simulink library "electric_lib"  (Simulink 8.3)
settings: Solver=ode45  StartTime=0.0  StopTime=10.0  RelTol=1e-3
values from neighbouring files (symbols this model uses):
  battery = class_REVS_battery    [class_REVS_electric.m]
  electric = class_REVS_electric(engine)    [electric_standard_car.m]
undefined symbols (not defined in the file or in its folder): alternator, converter, ConverterEfficiency_norm, emachine, starter
libraries: simulink x14, general_lib x14, audit_lib x9, electric_lib x5

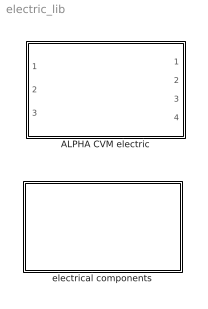
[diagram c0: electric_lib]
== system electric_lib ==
  ALPHA CVM electric : Subsystem  VariantControl=variants_electric_ALPHA
  electrical components : Subsystem

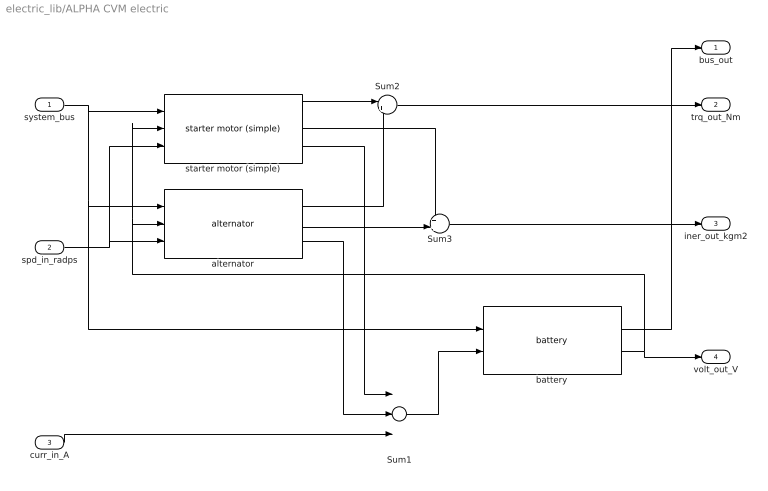
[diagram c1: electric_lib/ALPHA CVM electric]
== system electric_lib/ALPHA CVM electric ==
  system_bus : Inport
  spd_in_radps : Inport  Port=2
  curr_in_A : Inport  Port=3
  Sum1 : Sum  Inputs=+++
  Sum2 : Sum  Inputs=|++
  Sum3 : Sum  Inputs=++|
  alternator : electric_lib/electrical components/alternator  base_name=alternator  alternator=electric.alternator
  battery : electric_lib/electrical components/battery  BaseName=battery  battery=electric.battery
  starter motor (simple) : electric_lib/electrical components/starter motor (simple)  base_name=starter  starter=electric.starter
  bus_out : Outport
  trq_out_Nm : Outport  Port=2
  iner_out_kgm2 : Outport  Port=3
  volt_out_V : Outport  Port=4
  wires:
  spd_in_radps/1 -> alternator/3, starter motor (simple)/3
  Sum2/1 -> trq_out_Nm/1
  Sum3/1 -> iner_out_kgm2/1
  system_bus/1 -> battery/1, alternator/1, starter motor (simple)/1
  battery/2 -> volt_out_V/1, starter motor (simple)/2, alternator/2
  alternator/2 -> Sum3/2
  starter motor (simple)/2 -> Sum3/1
  alternator/1 -> Sum2/2
  starter motor (simple)/1 -> Sum2/1
  battery/1 -> bus_out/1
  starter motor (simple)/3 -> Sum1/1
  alternator/3 -> Sum1/2
  Sum1/1 -> battery/2
  curr_in_A/1 -> Sum1/3

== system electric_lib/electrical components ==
  alternator : Subsystem
  battery : Subsystem
  constant voltage power converter : Subsystem
  emachine : Subsystem
  starter motor (simple) : Subsystem
  thrushaft emachine : Subsystem
  variable voltage power converter : Subsystem

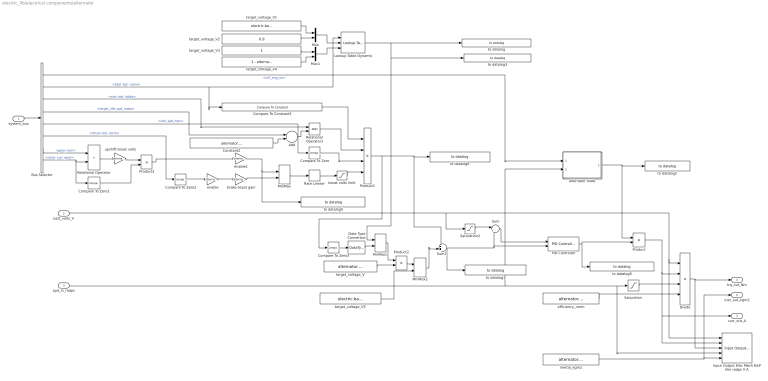
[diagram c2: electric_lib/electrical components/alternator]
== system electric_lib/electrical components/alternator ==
  system_bus : Inport
  batt_volts_V : Inport  Port=2
  spd_in_radps : Inport  Port=3
  Add : Sum
  Bus Selector : BusSelector  OutputSignals=powertrain.control.ctrl_eng_on,powertrain.signal4.batt_SoC_norm,powertrain.engine.eng_spd_radps,powertrain.engine.target_idle_spd_radps,vehicle.veh_spd_mps,driver.driver_brk_norm,powertrain.trans.ctrl.gear_num,powertrain.trans.ctrl.dct_core_ctrl.trans_curr_gear
  Compare To Constant2 : simulink/Logic and Bit Operations/Compare To Constant  relop=<=  const=alternator.regen_boost_max_battery_soc_norm  OutDataTypeStr=boolean  ZeroCross=off
  Compare To Zero{,1..3} (4 alike) : simulink/Logic and Bit Operations/Compare To Zero  relop=>  OutDataTypeStr=boolean  ZeroCross=off
  Constant2 : Constant  Value=alternator.regen_idle_speed_offset_radps
  Data Type Conversion : DataTypeConversion
  Divide : Product  Inputs=**//
  Input Output Elec Mech E&P Nm radps V A : audit_lib/Input Output Elec Mech E&P Nm radps V A  base_name=alternator  VerboseSignal=REVS.verbose
  Lookup Table Dynamic : simulink/Lookup Tables/Lookup Table Dynamic  LookUpMeth=Interpolation-Use End Values  OutDataTypeStr=double  OutputDataTypeScalingMode=Specify via dialog  OutDataType=fixdt('double')  OutScaling=2^-10  DoSatur=off
  MinMax : MinMax  Function=max  Inputs=2
  MinMax1 : MinMax  Function=max  Inputs=2
  MinMax2 : MinMax  Function=max  Inputs=2
  Mux : Mux  Inputs=2
  Mux1 : Mux  Inputs=2
  PID Controller : simulink/Continuous/PID Controller  Controller=PID  TimeDomain=Continuous-time  SampleTime=1  IntegratorMethod=Forward Euler  FilterMethod=Forward Euler  Form=Parallel  P=alternator.nominal_Kp * (1 + alternator.regen_Kp_multiplier*alternator.regen_enable)  I=alternator.nominal_Ki * (1 + alternator.regen_Ki_multiplier*alternator.regen_enable)  D=0  N=1  InitialConditionSource=internal  InitialConditionForIntegrator=0  InitialConditionForFilter=0  ExternalReset=falling  ZeroCross=off  LimitOutput=on  UpperSaturationLimit=0  LowerSaturationLimit=-alternator.max_current_A  LinearizeAsGain=on  AntiWindupMode=clamping  Kb=1  TrackingMode=off  Kt=1  PParamMin=[]  PParamMax=[]  IParamMin=[]  IParamMax=[]  DParamMin=[]  DParamMax=[]  NParamMin=[]  NParamMax=[]  KbParamMin=[]  KbParamMax=[]  KtParamMin=[]  KtParamMax=[]  POutMin=[]  POutMax=[]  IOutMin=[]  IOutMax=[]  DOutMin=[]  DOutMax=[]  NOutMin=[]  NOutMax=[]  KbOutMin=[]  KbOutMax=[]  KtOutMin=[]  KtOutMax=[]  IntegratorOutMin=[]  IntegratorOutMax=[]  FilterOutMin=[]  FilterOutMax=[]  SumOutMin=[]  SumOutMax=[]  SumI1OutMin=[]  SumI1OutMax=[]  SumI2OutMin=[]  SumI2OutMax=[]  SumI3OutMin=[]  SumI3OutMax=[]  SumDOutMin=[]  SumDOutMax=[]  SaturationOutMin=[]  SaturationOutMax=[]  IntegratorContinuousStateAttributes=''  IntegratorStateMustResolveToSignalObject=off  IntegratorRTWStateStorageClass=Auto  FilterContinuousStateAttributes=''  FilterStateMustResolveToSignalObject=off  FilterRTWStateStorageClass=Auto
  Product : Product
  Product1 : Product  Inputs=4
  Product2 : Product
  Product3 : Product
  Rate Limiter : RateLimiter  RisingSlewLimit=1/.15  FallingSlewLimit=-1/0.15  SampleTimeMode=inherited
  Relational Operator : RelationalOperator  Operator=>  OutDataTypeStr=boolean  ZeroCross=off
  Relational Operator1 : RelationalOperator  OutDataTypeStr=boolean  ZeroCross=off
  Saturation : Saturate  UpperLimit=Inf  LowerLimit=eps
  Saturation2 : Saturate  UpperLimit=Inf  LowerLimit=1  ZeroCross=off
  Sum : Sum  Inputs=|+-
  Sum1 : Sum  Inputs=++|
  alternator state : Subsystem
  boost volts limit : Saturate  UpperLimit=alternator.regen_max_boost_volts  LowerLimit=0  ZeroCross=off
  brake boost gain : Gain  Gain=alternator.regen_max_boost_volts
  efficiency_norm : Constant  Value=alternator.efficiency_norm
  enable : Gain  Gain=alternator.regen_enable
  enable1 : Gain  Gain=alternator.regen_enable
  inertia_kgm2 : Constant  Value=alternator.inertia_kgm2
  target_voltage_V : Constant  Value=alternator.target_voltage_V
  target_voltage_V1 : Constant  Value=electric.battery.initial_soc_norm
  target_voltage_V2 : Constant  Value=0.9
  target_voltage_V3 : Constant
  target_voltage_V4 : Constant  Value=1 - alternator.regen_enable
  target_voltage_V5 : Constant  Value=electric.battery.min_voltage_V
  to datalog : general_lib/to datalog  VarName=alternator.regen_SOC_state  WorkspaceName=datalog__alternator__regen_SOC_state  VerboseLevel=2  VerboseSignal=REVS.verbose
  to datalog1 : general_lib/to datalog  VarName=alternator.target_voltage  WorkspaceName=datalog__alternator__target_voltage  VerboseLevel=1  VerboseSignal=REVS.verbose
  to datalog2 : general_lib/to datalog  VarName=alternator.state  WorkspaceName=datalog__alternator__state  VerboseLevel=1  VerboseSignal=REVS.verbose
  to datalog3 : general_lib/to datalog  VarName=alternator.regen_state  WorkspaceName=datalog__alternator__regen_state  VerboseLevel=2  VerboseSignal=REVS.verbose
  to datalog5 : general_lib/to datalog  VarName=alternator.upshift_sig  WorkspaceName=datalog__alternator__upshift_sig  VerboseLevel=1  VerboseSignal=REVS.verbose
  to datalog6 : general_lib/to datalog  VarName=alternator.voltage_boost  WorkspaceName=datalog__alternator__voltage_boost  VerboseLevel=2  VerboseSignal=REVS.verbose
  to datalog8 : general_lib/to datalog  VarName=alternator.PID_current_A  WorkspaceName=datalog__alternator__PID_current_A  VerboseLevel=3  VerboseSignal=REVS.verbose
  upshift boost volts : Gain  Gain=alternator.regen_upshift_boost_volts
  trq_out_Nm : Outport
  iner_out_kgm2 : Outport  Port=2
  curr_out_A : Outport  Port=3
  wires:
  Constant2/1 -> Add/2
  Bus Selector/4 -> Add/1  "<target_idle_spd_radps>"
  Add/1 -> Relational Operator1/2
  Bus Selector/3 -> Relational Operator1/1  "<eng_spd_radps>"
  Lookup Table Dynamic/1 -> to datalog/1, to datalog3/1, MinMax1/1
  Bus Selector/1 -> alternator state/1(eng_on)  "<ctrl_eng_on>"
  Bus Selector/2 -> Lookup Table Dynamic/1, Compare To Constant2/1  "<batt_SoC_norm>"
  Compare To Zero/1 -> Product1/3
  Bus Selector/5 -> Compare To Zero/1  "<veh_spd_mps>"
  boost volts limit/1 -> Product1/4
  brake boost gain/1 -> MinMax/2
  Bus Selector/6 -> Compare To Zero2/1  "<driver_brk_norm>"
  Sum1/1 -> PID Controller/2, Sum/2, to datalog1/1
  batt_volts_V/1 -> Divide/1, Input Output Elec Mech E&P Nm radps V A/1, Saturation2/1
  target_voltage_V/1 -> Product2/2
  Product/1 -> Divide/2, curr_out_A/1, Input Output Elec Mech E&P Nm radps V A/2
  spd_in_radps/1 -> alternator state/2(spd_in_radps), Saturation/1, Input Output Elec Mech E&P Nm radps V A/4
  Saturation/1 -> Divide/3
  efficiency_norm/1 -> Divide/4
  Divide/1 -> Input Output Elec Mech E&P Nm radps V A/3, trq_out_Nm/1
  inertia_kgm2/1 -> iner_out_kgm2/1, Input Output Elec Mech E&P Nm radps V A/5
  Saturation2/1 -> Sum/1
  alternator state/1(state) -> to datalog2/1, Product/1
  system_bus/1 -> Bus Selector/1
  Compare To Constant2/1 -> Product1/1
  Bus Selector/7 -> Relational Operator/1  "<gear_num>"
  Bus Selector/8 -> Compare To Zero1/1, Relational Operator/2  "<trans_curr_gear>"
  Relational Operator/1 -> upshift boost volts/1
  Product3/1 -> enable1/1
  MinMax/1 -> Rate Limiter/1
  PID Controller/1 -> Product/2, to datalog8/1
  Relational Operator1/1 -> Product1/2
  enable1/1 -> to datalog5/1, MinMax/1
  upshift boost volts/1 -> Product3/1
  Compare To Zero1/1 -> Product3/2
  Compare To Zero2/1 -> enable/1
  enable/1 -> brake boost gain/1
  target_voltage_V1/1 -> Mux/1
  target_voltage_V2/1 -> Mux/2
  Mux/1 -> Lookup Table Dynamic/2
  target_voltage_V3/1 -> Mux1/1
  target_voltage_V4/1 -> Mux1/2
  Mux1/1 -> Lookup Table Dynamic/3
  Product1/1 -> Sum1/1, to datalog6/1, Compare To Zero3/1
  Sum/1 -> PID Controller/1
  MinMax2/1 -> Sum1/2
  Compare To Zero3/1 -> Data Type Conversion/1
  Data Type Conversion/1 -> MinMax1/2
  MinMax1/1 -> Product2/1
  Product2/1 -> MinMax2/1
  target_voltage_V5/1 -> MinMax2/2
  Rate Limiter/1 -> boost volts limit/1

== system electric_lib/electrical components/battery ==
  note: thermal model will eventually be a variant, probably, with a "simple" thermal model version
  system_bus : Inport
  curr_out_A : Inport  Port=2
  Bus Creator : BusCreator  Inputs=6
  Bus Selector : BusSelector  OutputSignals=ambient.temp_degC
  Elec E&P V A Standalone : audit_lib/Elec E&P V A Standalone  base_name=battery  VerboseSignal=REVS.verbose
  Gain : Gain  Gain=-1
  Memory2 : Memory
  battery power limits : Subsystem
  dynamic battery model : Subsystem
  thermal model : Subsystem
  bus_out : Outport
  volts_out_V : Outport  Port=2
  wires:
  thermal model/1(batt_temp_degC) -> Bus Creator/1, battery power limits/1(batt_temp_degC), dynamic battery model/1(batt_temp_degC)  "batt_temp_degC"
  Bus Selector/1 -> thermal model/2(amb_temp_degC)  "<temp_degC>"
  dynamic battery model/1(SoC_norm) -> battery power limits/2(SoC_norm), Bus Creator/2  "batt_SoC_norm"
  dynamic battery model/5(chg_res_Ohm) -> battery power limits/6(chg_res_Ohms)
  dynamic battery model/4(dis_res_Ohm) -> battery power limits/5(dis_res_Ohms)
  dynamic battery model/2(OCV_V) -> battery power limits/3(OCV_V)
  battery power limits/1(max_dis_pwr_W) -> Bus Creator/3  "batt_max_dis_pwr_W"
  battery power limits/2(max_chg_pwr_W) -> Bus Creator/4  "batt_max_chg_pwr_W"
  curr_out_A/1 -> Gain/1, Memory2/1  "batt_curr_A"
  Bus Creator/1 -> bus_out/1
  Gain/1 -> Elec E&P V A Standalone/2
  dynamic battery model/6(loss_pwr_W) -> thermal model/1(loss_pwr_W)
  system_bus/1 -> Bus Selector/1
  dynamic battery model/3(volts_out_V) -> Elec E&P V A Standalone/1, volts_out_V/1, Bus Creator/6, battery power limits/4(volts_out_V)  "batt_volts_V"
  Memory2/1 -> dynamic battery model/2(curr_out_A), Bus Creator/5  "batt_curr_A"

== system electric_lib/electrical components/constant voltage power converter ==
  volts_in_V : Inport
  curr_out_A : Inport  Port=2
  Constant2 : Constant  Value=converter.output_voltage_V
  variable voltage power converter : electric_lib/electrical components/variable voltage power converter  AuditBaseName=low_voltage_DCDC  ConverterEfficiency_norm=converter.efficiency_norm
  bus_out : Outport
  volts_out_V : Outport  Port=2
  curr_in_A : Outport  Port=3
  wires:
  variable voltage power converter/3 -> curr_in_A/1
  variable voltage power converter/1 -> bus_out/1
  variable voltage power converter/2 -> volts_out_V/1
  volts_in_V/1 -> variable voltage power converter/2
  curr_out_A/1 -> variable voltage power converter/3
  Constant2/1 -> variable voltage power converter/1

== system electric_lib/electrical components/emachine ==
  system_bus : Inport
  spd_out_radps : Inport  Port=2
  voltage_bus : Inport  Port=3
  Terminator : Terminator
  thrushaft emachine : electric_lib/electrical components/thrushaft emachine  EMachineBaseName=drive_motor  OutputSignals=drive_motor_enable,drive_motor_trq_rqst_nm  emachine=emachine_struct_name
  zero : Constant  Value=0
  bus_out : Outport
  trq_out_Nm : Outport  Port=2
  iner_out_kgm2 : Outport  Port=3
  current_bus : Outport  Port=4
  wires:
  zero/1 -> thrushaft emachine/2, thrushaft emachine/3
  system_bus/1 -> thrushaft emachine/1
  thrushaft emachine/1 -> bus_out/1
  thrushaft emachine/2 -> trq_out_Nm/1
  thrushaft emachine/3 -> iner_out_kgm2/1
  thrushaft emachine/5 -> current_bus/1
  spd_out_radps/1 -> thrushaft emachine/4
  voltage_bus/1 -> thrushaft emachine/5
  thrushaft emachine/4 -> Terminator/1

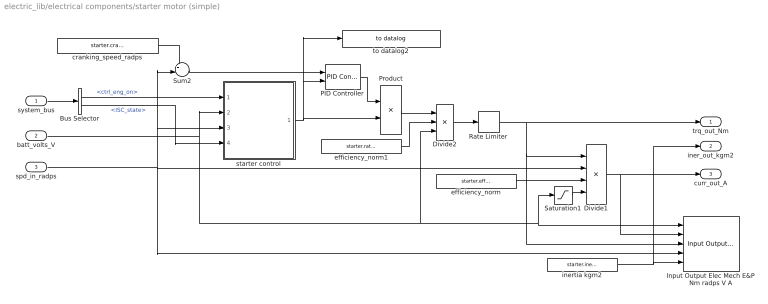
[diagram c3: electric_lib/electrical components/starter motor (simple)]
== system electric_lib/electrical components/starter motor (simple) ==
  system_bus : Inport
  batt_volts_V : Inport  Port=2
  spd_in_radps : Inport  Port=3
  Bus Selector : BusSelector  OutputSignals=powertrain.control.ctrl_eng_on,powertrain.engine.ISC_state
  Divide1 : Product  Inputs=**//
  Divide2 : Product  Inputs=*/*
  Input Output Elec Mech E&P Nm radps V A : audit_lib/Input Output Elec Mech E&P Nm radps V A  base_name=starter  VerboseSignal=REVS.verbose
  PID Controller : simulink/Continuous/PID Controller  Controller=PID  TimeDomain=Continuous-time  SampleTime=1  IntegratorMethod=Forward Euler  FilterMethod=Forward Euler  Form=Parallel  P=10  I=10  D=0  N=1  InitialConditionSource=internal  InitialConditionForIntegrator=0  InitialConditionForFilter=0  ExternalReset=rising  ZeroCross=off  LimitOutput=on  UpperSaturationLimit=starter.max_torque_Nm  LowerSaturationLimit=0  LinearizeAsGain=on  AntiWindupMode=none  Kb=1  TrackingMode=off  Kt=1  PParamMin=[]  PParamMax=[]  IParamMin=[]  IParamMax=[]  DParamMin=[]  DParamMax=[]  NParamMin=[]  NParamMax=[]  KbParamMin=[]  KbParamMax=[]  KtParamMin=[]  KtParamMax=[]  POutMin=[]  POutMax=[]  IOutMin=[]  IOutMax=[]  DOutMin=[]  DOutMax=[]  NOutMin=[]  NOutMax=[]  KbOutMin=[]  KbOutMax=[]  KtOutMin=[]  KtOutMax=[]  IntegratorOutMin=[]  IntegratorOutMax=[]  FilterOutMin=[]  FilterOutMax=[]  SumOutMin=[]  SumOutMax=[]  SumI1OutMin=[]  SumI1OutMax=[]  SumI2OutMin=[]  SumI2OutMax=[]  SumI3OutMin=[]  SumI3OutMax=[]  SumDOutMin=[]  SumDOutMax=[]  SaturationOutMin=[]  SaturationOutMax=[]  IntegratorContinuousStateAttributes=''  IntegratorStateMustResolveToSignalObject=off  IntegratorRTWStateStorageClass=Auto  FilterContinuousStateAttributes=''  FilterStateMustResolveToSignalObject=off  FilterRTWStateStorageClass=Auto
  Product : Product
  Rate Limiter : RateLimiter  RisingSlewLimit=electric.starter.max_torque_Nm * 10  FallingSlewLimit=-electric.starter.max_torque_Nm * 10  SampleTimeMode=inherited
  Saturation1 : Saturate  UpperLimit=Inf  LowerLimit=eps
  Sum2 : Sum  Inputs=+-|
  cranking_speed_radps : Constant  Value=starter.cranking_speed_radps
  efficiency_norm : Constant  Value=starter.efficiency_norm
  efficiency_norm1 : Constant  Value=starter.rated_voltage_V
  inertia kgm2 : Constant  Value=starter.inertia_kgm2
  starter control : Subsystem
  to datalog2 : general_lib/to datalog  VarName=electric.starter_state  WorkspaceName=datalog__electric__starter_state  VerboseLevel=3  VerboseSignal=REVS.verbose
  trq_out_Nm : Outport
  iner_out_kgm2 : Outport  Port=2
  curr_out_A : Outport  Port=3
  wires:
  Bus Selector/2 -> starter control/4(ISC_state)  "<ISC_state>"
  Rate Limiter/1 -> trq_out_Nm/1, Divide1/1, Input Output Elec Mech E&P Nm radps V A/3
  inertia kgm2/1 -> Input Output Elec Mech E&P Nm radps V A/5, iner_out_kgm2/1
  Divide2/1 -> Rate Limiter/1
  spd_in_radps/1 -> Divide1/2, Input Output Elec Mech E&P Nm radps V A/4, Sum2/2, starter control/3(spd_in_radps)
  batt_volts_V/1 -> starter control/2(batt_volts_V), Saturation1/1, Input Output Elec Mech E&P Nm radps V A/1, Divide2/3
  efficiency_norm/1 -> Divide1/3
  Saturation1/1 -> Divide1/4
  cranking_speed_radps/1 -> Sum2/1
  Sum2/1 -> PID Controller/1
  PID Controller/1 -> Product/1
  starter control/1(state) -> Product/2, to datalog2/1, PID Controller/2
  system_bus/1 -> Bus Selector/1
  Bus Selector/1 -> starter control/1(eng_on)  "<ctrl_eng_on>"
  Divide1/1 -> curr_out_A/1, Input Output Elec Mech E&P Nm radps V A/2
  Product/1 -> Divide2/1
  efficiency_norm1/1 -> Divide2/2

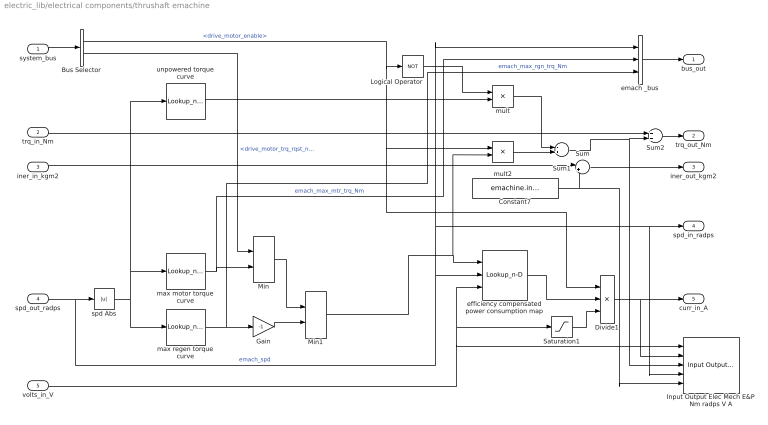
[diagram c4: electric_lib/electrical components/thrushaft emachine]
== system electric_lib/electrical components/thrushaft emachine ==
  system_bus : Inport
  trq_in_Nm : Inport  Port=2
  iner_in_kgm2 : Inport  Port=3
  spd_out_radps : Inport  Port=4
  volts_in_V : Inport  Port=5
  Bus Selector : BusSelector  OutputSignals=drive_motor_enable,drive_motor_trq_rqst_nm
  Constant7 : Constant  Value=emachine.inertia_kgm2
  Divide1 : Product  Inputs=**/
  Gain : Gain  Gain=-1
  Input Output Elec Mech E&P Nm radps V A : audit_lib/Input Output Elec Mech E&P Nm radps V A  base_name=drive_motor  VerboseSignal=REVS.verbose
  Logical Operator : Logic  Operator=NOT  AllPortsSameDT=off  OutDataTypeStr=boolean
  Min : MinMax  Inputs=2
  Min1 : MinMax  Function=max  Inputs=2
  Saturation1 : Saturate  UpperLimit=Inf  LowerLimit=eps  ZeroCross=off
  Sum : Sum  Inputs=|++
  Sum1 : Sum  Inputs=-+
  Sum2 : Sum
  efficiency compensated power consumption map : Lookup_n-D  NumberOfTableDimensions=3  BreakpointsForDimension1=emachine.power_map_torque_index_Nm  BreakpointsForDimension2=emachine.power_map_speed_index_radps  BreakpointsForDimension3=emachine.power_map_voltage_index_V  IndexSearchMethod=Linear search  BeginIndexSearchUsingPreviousIndexResult=on  Table=emachine.power_map_W  ExtrapMethod=Clip  UseLastTableValue=on  RndMeth=Simplest
  emach _bus : BusCreator  Inputs=3
  max motor torque curve : Lookup_n-D  NumberOfTableDimensions=1  BreakpointsForDimension1=emachine.max_torque_curve_speed_radps  BeginIndexSearchUsingPreviousIndexResult=on  Table=emachine.max_motor_torque_curve_Nm  ExtrapMethod=Clip  UseLastTableValue=on  RndMeth=Simplest
  max regen torque curve : Lookup_n-D  NumberOfTableDimensions=1  BreakpointsForDimension1=emachine.max_torque_curve_speed_radps  BeginIndexSearchUsingPreviousIndexResult=on  Table=emachine.max_regen_torque_curve_Nm  ExtrapMethod=Clip  UseLastTableValue=on  RndMeth=Simplest
  mult : Product
  mult2 : Product
  spd Abs : Abs  ZeroCross=off
  unpowered torque curve : Lookup_n-D  NumberOfTableDimensions=1  BreakpointsForDimension1=emachine.spinloss_speed_radps  BeginIndexSearchUsingPreviousIndexResult=on  Table=emachine.spinloss_torque_Nm  ExtrapMethod=Clip  UseLastTableValue=on  RndMeth=Simplest
  bus_out : Outport
  trq_out_Nm : Outport  Port=2
  iner_out_kgm2 : Outport  Port=3
  spd_in_radps : Outport  Port=4
  curr_in_A : Outport  Port=5
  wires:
  Sum1/1 -> Sum2/2, Input Output Elec Mech E&P Nm radps V A/3
  volts_in_V/1 -> Saturation1/1, efficiency compensated power consumption map/3, Input Output Elec Mech E&P Nm radps V A/1
  efficiency compensated power consumption map/1 -> Divide1/2
  system_bus/1 -> Bus Selector/1
  Bus Selector/1 -> mult2/1, Divide1/1, Logical Operator/1  "<drive_motor_enable>"
  Logical Operator/1 -> mult/1
  mult/1 -> Sum1/1
  mult2/1 -> Sum1/2
  unpowered torque curve/1 -> mult/2
  spd Abs/1 -> max regen torque curve/1, max motor torque curve/1, unpowered torque curve/1
  Min1/1 -> efficiency compensated power consumption map/1, mult2/2
  max motor torque curve/1 -> Min/2, emach _bus/2  "emach_max_mtr_trq_Nm"
  trq_in_Nm/1 -> Sum2/1
  Sum2/1 -> trq_out_Nm/1
  iner_in_kgm2/1 -> Sum/1
  Constant7/1 -> Sum/2, Input Output Elec Mech E&P Nm radps V A/5
  Sum/1 -> iner_out_kgm2/1
  Bus Selector/2 -> Min/1  "<drive_motor_trq_rqst_nm>"
  Divide1/1 -> curr_in_A/1, Input Output Elec Mech E&P Nm radps V A/2
  Saturation1/1 -> Divide1/3
  spd_out_radps/1 -> efficiency compensated power consumption map/2, emach _bus/1, Input Output Elec Mech E&P Nm radps V A/4, spd_in_radps/1, spd Abs/1  "emach_spd"
  emach _bus/1 -> bus_out/1
  max regen torque curve/1 -> Gain/1, emach _bus/3  "emach_max_rgn_trq_Nm"
  Min/1 -> Min1/1
  Gain/1 -> Min1/2

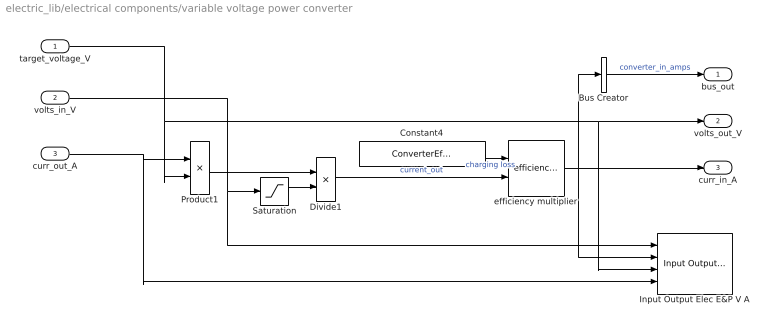
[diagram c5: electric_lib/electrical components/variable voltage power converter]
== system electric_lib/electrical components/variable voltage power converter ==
  target_voltage_V : Inport
  volts_in_V : Inport  Port=2
  curr_out_A : Inport  Port=3
  Bus Creator : BusCreator  Inputs=1
  Constant4 : Constant  Value=ConverterEfficiency_norm
  Divide1 : Product  Inputs=*/
  Input Output Elec E&P V A : audit_lib/Input Output Elec E&P V A  base_name=econverter  VerboseSignal=REVS.verbose
  Product1 : Product
  Saturation : Saturate  UpperLimit=Inf  LowerLimit=eps
  efficiency multiplier : general_lib/efficiency multiplier  MultiplyPosInputs=false
  bus_out : Outport
  volts_out_V : Outport  Port=2
  curr_in_A : Outport  Port=3
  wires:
  Constant4/1 -> efficiency multiplier/1  "charging loss"
  efficiency multiplier/1 -> Input Output Elec E&P V A/2, curr_in_A/1, Bus Creator/1
  Divide1/1 -> efficiency multiplier/2  "current_out"
  Saturation/1 -> Divide1/2
  Product1/1 -> Divide1/1
  volts_in_V/1 -> Input Output Elec E&P V A/1, Saturation/1
  curr_out_A/1 -> Input Output Elec E&P V A/4, Product1/1
  Bus Creator/1 -> bus_out/1  "converter_in_amps"
  target_voltage_V/1 -> Input Output Elec E&P V A/3, volts_out_V/1, Product1/2

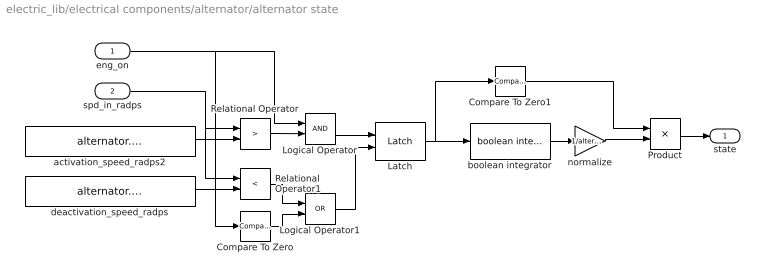
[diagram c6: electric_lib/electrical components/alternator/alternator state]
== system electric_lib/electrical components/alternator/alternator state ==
  eng_on : Inport
  spd_in_radps : Inport  Port=2
  Compare To Zero : simulink/Logic and Bit Operations/Compare To Zero  relop===  OutDataTypeStr=boolean
  Compare To Zero1 : simulink/Logic and Bit Operations/Compare To Zero  relop=>  OutDataTypeStr=boolean
  Latch : general_lib/Latch  tb=Off  InitialCondition=0
  Logical Operator : Logic  AllPortsSameDT=off  OutDataTypeStr=boolean
  Logical Operator1 : Logic  Operator=OR  AllPortsSameDT=off  OutDataTypeStr=boolean
  Product : Product
  Relational Operator : RelationalOperator  Operator=>  OutDataTypeStr=boolean
  Relational Operator1 : RelationalOperator  Operator=<  OutDataTypeStr=boolean
  activation_speed_radps2 : Constant  Value=alternator.activate_speed_radps
  boolean integrator : general_lib/boolean integrator  UpperSaturationLimit=alternator.activation_time_secs
  deactivation_speed_radps : Constant  Value=alternator.deactivate_speed_radps
  normalize : Gain  Gain=1/alternator.activation_time_secs
  state : Outport
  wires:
  Relational Operator/1 -> Logical Operator/2
  spd_in_radps/1 -> Relational Operator/1, Relational Operator1/1
  activation_speed_radps2/1 -> Relational Operator/2
  Logical Operator1/1 -> Latch/2
  Logical Operator/1 -> Latch/1
  deactivation_speed_radps/1 -> Relational Operator1/2
  Latch/1 -> Compare To Zero1/1, boolean integrator/1
  Relational Operator1/1 -> Logical Operator1/1
  Compare To Zero/1 -> Logical Operator1/2
  Product/1 -> state/1
  boolean integrator/1 -> normalize/1
  Compare To Zero1/1 -> Product/1
  eng_on/1 -> Compare To Zero/1, Logical Operator/1
  normalize/1 -> Product/2

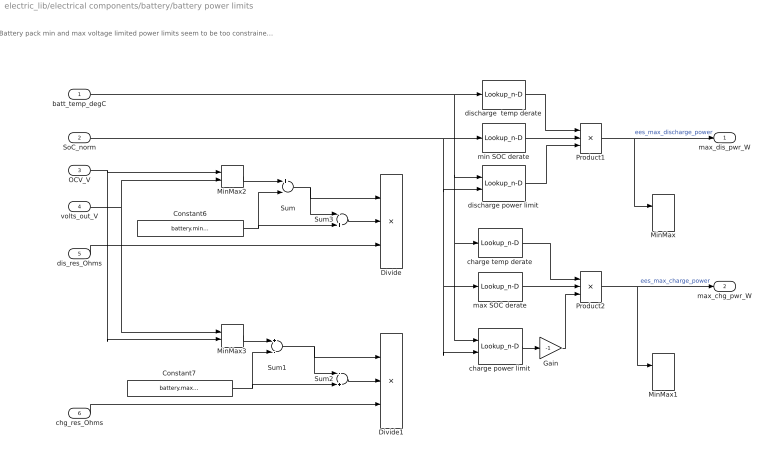
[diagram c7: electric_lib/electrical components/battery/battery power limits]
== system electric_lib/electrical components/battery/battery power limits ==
  note: Battery pack min and max voltage limited power limits seem to be too constrained compared with actual pack capacity so either the calculated limits are too low or the source data is overly conservative... so they are disabled for now until further investigation
  batt_temp_degC : Inport
  SoC_norm : Inport  Port=2
  OCV_V : Inport  Port=3
  volts_out_V : Inport  Port=4
  dis_res_Ohms : Inport  Port=5
  chg_res_Ohms : Inport  Port=6
  Constant6 : Constant  Value=battery.min_voltage_V
  Constant7 : Constant  Value=battery.max_voltage_V
  Divide : Product  Inputs=**/
  Divide1 : Product  Inputs=**/
  Gain : Gain  Gain=-1
  MinMax : MinMax  Inputs=2
  MinMax1 : MinMax  Function=max  Inputs=2
  MinMax2 : MinMax  Inputs=2
  MinMax3 : MinMax  Inputs=2
  Product1 : Product  Inputs=3
  Product2 : Product  Inputs=3
  Sum : Sum  Inputs=+-
  Sum1 : Sum  Inputs=+-
  Sum2 : Sum  Inputs=-+
  Sum3 : Sum  Inputs=-+
  charge power limit : Lookup_n-D  BreakpointsForDimension1=battery.powerlimit_map_index_temp_degC  BreakpointsForDimension2=battery.powerlimit_map_index_soc_norm  Table=battery.powerlimit_charge_map_W  RndMeth=Simplest
  charge temp derate : Lookup_n-D  NumberOfTableDimensions=1  BreakpointsForDimension1=battery.temperature_power_derate_index_temp_degC  IndexSearchMethod=Linear search  BeginIndexSearchUsingPreviousIndexResult=on  Table=battery.temperature_power_charge_derate_norm  ExtrapMethod=Clip  RndMeth=Simplest
  discharge  temp derate : Lookup_n-D  NumberOfTableDimensions=1  BreakpointsForDimension1=battery.temperature_power_derate_index_temp_degC  IndexSearchMethod=Linear search  BeginIndexSearchUsingPreviousIndexResult=on  Table=battery.temperature_power_discharge_derate_norm  ExtrapMethod=Clip  RndMeth=Simplest
  discharge power limit : Lookup_n-D  BreakpointsForDimension1=battery.powerlimit_map_index_temp_degC  BreakpointsForDimension2=battery.powerlimit_map_index_soc_norm  Table=battery.powerlimit_discharge_map_W  RndMeth=Simplest
  max SOC derate : Lookup_n-D  NumberOfTableDimensions=1  BreakpointsForDimension1=battery.charge_derate_soc_norm  IndexSearchMethod=Linear search  BeginIndexSearchUsingPreviousIndexResult=on  Table=[1 0]  ExtrapMethod=Clip  RndMeth=Simplest
  min SOC derate : Lookup_n-D  NumberOfTableDimensions=1  BreakpointsForDimension1=battery.discharge_derate_soc_norm  IndexSearchMethod=Linear search  BeginIndexSearchUsingPreviousIndexResult=on  Table=[0 1]  ExtrapMethod=Clip  RndMeth=Simplest
  max_dis_pwr_W : Outport
  max_chg_pwr_W : Outport  Port=2
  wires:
  Sum3/1 -> Divide/2
  Sum2/1 -> Divide1/2
  volts_out_V/1 -> MinMax3/1, MinMax2/2
  MinMax2/1 -> Sum/1
  MinMax3/1 -> Sum1/1
  OCV_V/1 -> MinMax3/2, MinMax2/1
  Gain/1 -> Product2/3
  Constant6/1 -> Sum/2, Sum3/2
  batt_temp_degC/1 -> discharge  temp derate/1, discharge power limit/1, charge power limit/1, charge temp derate/1
  dis_res_Ohms/1 -> Divide/3
  chg_res_Ohms/1 -> Divide1/3
  Divide/1 -> ?
  Sum1/1 -> Sum2/1, Divide1/1
  Constant7/1 -> Sum1/2, Sum2/2
  discharge  temp derate/1 -> Product1/1
  discharge power limit/1 -> Product1/3
  charge power limit/1 -> Gain/1
  Divide1/1 -> ?
  max SOC derate/1 -> Product2/2
  Sum/1 -> Sum3/1, Divide/1
  min SOC derate/1 -> Product1/2
  Product2/1 -> max_chg_pwr_W/1, MinMax1/1  "ees_max_charge_power"
  SoC_norm/1 -> min SOC derate/1, discharge power limit/2, charge power limit/2, max SOC derate/1
  charge temp derate/1 -> Product2/1
  Product1/1 -> MinMax/1, max_dis_pwr_W/1  "ees_max_discharge_power"
  ? -> MinMax/2
  ? -> MinMax1/2

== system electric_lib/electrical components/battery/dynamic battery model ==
  batt_temp_degC : Inport
  curr_out_A : Inport  Port=2
  SOC : Subsystem
  dynamic voltage / loss model : Subsystem
  SoC_norm : Outport
  OCV_V : Outport  Port=2
  volts_out_V : Outport  Port=3
  dis_res_Ohm : Outport  Port=4
  chg_res_Ohm : Outport  Port=5
  loss_pwr_W : Outport  Port=6
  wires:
  SOC/3(pile_curr_A) -> dynamic voltage / loss model/5(pile_curr_A)
  curr_out_A/1 -> SOC/1(batt_curr_A), dynamic voltage / loss model/1(batt_curr_A)
  dynamic voltage / loss model/4(chg_res_Ohm) -> chg_res_Ohm/1
  dynamic voltage / loss model/3(dis_res_Ohm) -> dis_res_Ohm/1
  SOC/1(SoC_norm) -> SoC_norm/1, dynamic voltage / loss model/2(SoC_norm)
  dynamic voltage / loss model/2(batt_volts_V) -> volts_out_V/1
  dynamic voltage / loss model/1(OCV_V) -> OCV_V/1
  SOC/2(chg_eff_norm) -> dynamic voltage / loss model/4(chg_eff_norm)
  batt_temp_degC/1 -> dynamic voltage / loss model/3(batt_temp_degC), SOC/2(batt_temp_degC)
  dynamic voltage / loss model/5(loss_pwr_W) -> loss_pwr_W/1

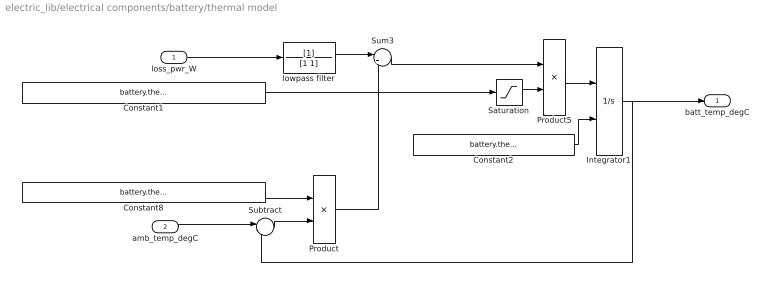
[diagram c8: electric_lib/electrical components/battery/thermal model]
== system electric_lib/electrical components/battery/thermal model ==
  loss_pwr_W : Inport
  amb_temp_degC : Inport  Port=2
  Constant1 : Constant  Value=battery.thermal.pack_heat_capacity_JpK
  Constant2 : Constant  Value=battery.thermal.initial_temp_degC
  Constant8 : Constant  Value=battery.thermal.pack_total_conductance_WpK
  Integrator1 : Integrator  InitialConditionSource=external
  Product : Product
  Product5 : Product  Inputs=*/
  Saturation : Saturate  UpperLimit=Inf  LowerLimit=eps
  Subtract : Sum  Inputs=|-+
  Sum3 : Sum  Inputs=|+-
  lowpass filter : TransferFcn  Denominator=[1 1]
  batt_temp_degC : Outport
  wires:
  lowpass filter/1 -> Sum3/1
  loss_pwr_W/1 -> lowpass filter/1
  Product5/1 -> Integrator1/1
  Sum3/1 -> Product5/1
  Integrator1/1 -> Subtract/2, batt_temp_degC/1
  Product/1 -> Sum3/2
  Saturation/1 -> Product5/2
  Subtract/1 -> Product/2
  amb_temp_degC/1 -> Subtract/1
  Constant1/1 -> Saturation/1
  Constant8/1 -> Product/1
  Constant2/1 -> Integrator1/2

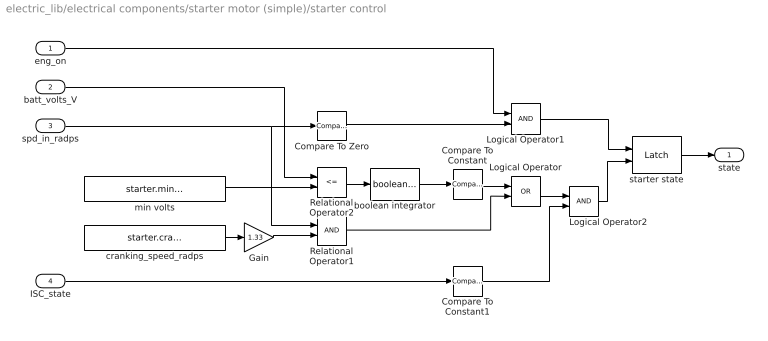
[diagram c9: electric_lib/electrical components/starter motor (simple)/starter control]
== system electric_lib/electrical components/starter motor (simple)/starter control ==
  eng_on : Inport
  batt_volts_V : Inport  Port=2
  spd_in_radps : Inport  Port=3
  ISC_state : Inport  Port=4
  Compare To Constant : simulink/Logic and Bit Operations/Compare To Constant  relop=>=  const=1  OutDataTypeStr=boolean
  Compare To Constant1 : simulink/Logic and Bit Operations/Compare To Constant  relop=~=  const=0  OutDataTypeStr=boolean
  Compare To Zero : simulink/Logic and Bit Operations/Compare To Zero  relop===  OutDataTypeStr=boolean
  Gain : Gain  Gain=1.33
  Logical Operator : Logic  Operator=OR  AllPortsSameDT=off  OutDataTypeStr=boolean
  Logical Operator1 : Logic  AllPortsSameDT=off  OutDataTypeStr=boolean
  Logical Operator2 : Logic  AllPortsSameDT=off  OutDataTypeStr=boolean
  Relational Operator1 : RelationalOperator  OutDataTypeStr=boolean
  Relational Operator2 : RelationalOperator  Operator=<=  OutDataTypeStr=boolean
  boolean integrator : general_lib/boolean integrator  UpperSaturationLimit=0.25  Normalize=on
  cranking_speed_radps : Constant  Value=starter.cranking_speed_radps
  min volts : Constant  Value=starter.min_voltage_V
  starter state : general_lib/Latch  tb=Off  InitialCondition=0
  state : Outport
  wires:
  ISC_state/1 -> Compare To Constant1/1
  Compare To Constant1/1 -> Logical Operator2/2
  Logical Operator2/1 -> starter state/2
  Logical Operator/1 -> Logical Operator2/1
  min volts/1 -> Relational Operator2/2
  Relational Operator2/1 -> boolean integrator/1
  Compare To Zero/1 -> Logical Operator1/2
  starter state/1 -> state/1
  Relational Operator1/1 -> Logical Operator/2
  Gain/1 -> Relational Operator1/2
  spd_in_radps/1 -> Compare To Zero/1, Relational Operator1/1
  batt_volts_V/1 -> Relational Operator2/1
  cranking_speed_radps/1 -> Gain/1
  Logical Operator1/1 -> starter state/1
  eng_on/1 -> Logical Operator1/1
  boolean integrator/1 -> Compare To Constant/1
  Compare To Constant/1 -> Logical Operator/1

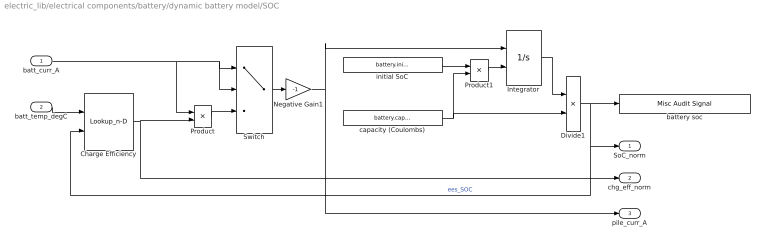
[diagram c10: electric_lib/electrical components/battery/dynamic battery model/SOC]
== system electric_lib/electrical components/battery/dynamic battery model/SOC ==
  batt_curr_A : Inport
  batt_temp_degC : Inport  Port=2
  Charge Efficiency : Lookup_n-D  BreakpointsForDimension1=battery.charge_efficiency_index_temp_degC  BreakpointsForDimension2=battery.charge_efficiency_index_soc_norm  Table=battery.charge_efficiency_map_norm  RndMeth=Simplest  MaximumIndicesForEachDimension=battery.open_circuit_voltage_map_charge_V_size
  Divide1 : Product  Inputs=*/
  Integrator : Integrator  InitialConditionSource=external  InitialCondition=battery.initial_soc_norm * battery.capacity_Coulombs  LimitOutput=on  UpperSaturationLimit=battery.capacity_Coulombs  LowerSaturationLimit=0
  Negative Gain1 : Gain  Gain=-1
  Product : Product
  Product1 : Product
  Switch : Switch  OutDataTypeStr=double
  battery soc : audit_lib/Misc Audit Signal  AuditBase=Electrical  VarName=battery_SoC_norm  BaseName=''  WorkspaceName=audit__elec__battery_SoC_norm  VerboseSignal=REVS.verbose
  capacity (Coulombs) : Constant  Value=battery.capacity_Coulombs
  initial SoC : Constant  Value=battery.initial_soc_norm
  SoC_norm : Outport
  chg_eff_norm : Outport  Port=2
  pile_curr_A : Outport  Port=3
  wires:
  Charge Efficiency/1 -> chg_eff_norm/1, Product/2
  Negative Gain1/1 -> Integrator/1, pile_curr_A/1
  Product/1 -> Switch/3
  Switch/1 -> Negative Gain1/1
  batt_curr_A/1 -> Switch/2, Switch/1, Product/1
  batt_temp_degC/1 -> Charge Efficiency/1
  Integrator/1 -> Divide1/1
  capacity (Coulombs)/1 -> Product1/2, Divide1/2
  Divide1/1 -> battery soc/1, Charge Efficiency/2, SoC_norm/1  "ees_SOC"
  Product1/1 -> Integrator/2
  initial SoC/1 -> Product1/1

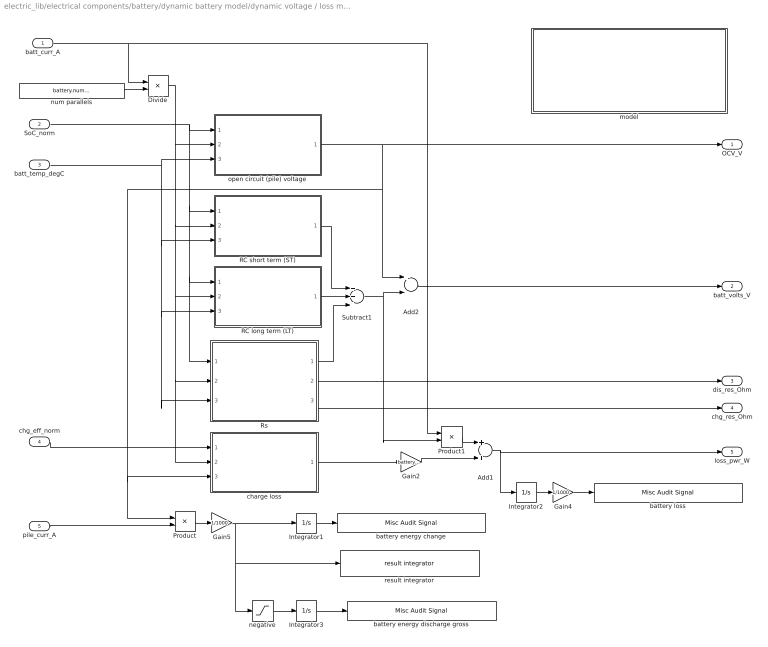
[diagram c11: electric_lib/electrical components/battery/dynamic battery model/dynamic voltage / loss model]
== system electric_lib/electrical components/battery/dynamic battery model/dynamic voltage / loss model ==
  batt_curr_A : Inport
  SoC_norm : Inport  Port=2
  batt_temp_degC : Inport  Port=3
  chg_eff_norm : Inport  Port=4
  pile_curr_A : Inport  Port=5
  Add1 : Sum
  Add2 : Sum  Inputs=+-
  Divide : Product  Inputs=*/
  Gain2 : Gain  Gain=battery.num_parallel_cells
  Gain4 : Gain  Gain=1/1000
  Gain5 : Gain  Gain=1/1000
  Integrator1 : Integrator  ZeroCross=off
  Integrator2 : Integrator  ZeroCross=off
  Integrator3 : Integrator  ZeroCross=off
  Product : Product
  Product1 : Product
  RC long term (LT) : Subsystem
  RC short term (ST) : Subsystem
  Rs : Subsystem
  Subtract1 : Sum  Inputs=+++
  battery energy change : audit_lib/Misc Audit Signal  AuditBase=Electrical  VarName=battery_energy_delta_kJ  BaseName=''  WorkspaceName=audit__elec__battery_energy_delta_kJ  VerboseSignal=REVS.verbose
  battery energy discharge gross : audit_lib/Misc Audit Signal  AuditBase=Electrical  VarName=battery_discharge_gross_kJ  BaseName=''  WorkspaceName=audit__elec__battery_discharge_gross_kJ  VerboseSignal=REVS.verbose
  battery loss : audit_lib/Misc Audit Signal  AuditBase=Electrical  VarName=battery_loss_kJ  BaseName=''  WorkspaceName=audit__elec__battery_loss_kJ  VerboseSignal=REVS.verbose
  charge loss : Subsystem
  model : Subsystem
  negative : Saturate  UpperLimit=0  LowerLimit=-Inf
  num parallels : Constant  Value=battery.num_parallel_cells
  open circuit (pile) voltage : Subsystem
  result integrator : general_lib/result integrator  ResultSignalName=energy_delta_kJ  ResultBaseName=BaseName
  OCV_V : Outport
  batt_volts_V : Outport  Port=2
  dis_res_Ohm : Outport  Port=3
  chg_res_Ohm : Outport  Port=4
  loss_pwr_W : Outport  Port=5
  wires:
  Gain4/1 -> battery loss/1
  Product1/1 -> Add1/1
  Gain2/1 -> Add1/2
  Integrator2/1 -> Gain4/1
  batt_curr_A/1 -> Product1/1, Divide/1
  num parallels/1 -> Divide/2
  Divide/1 -> RC short term (ST)/2(cell_curr_A), RC long term (LT)/2(cell_curr_A), Rs/2(cell_curr_A), charge loss/2(cell_curr_A), open circuit (pile) voltage/2(cell_curr_A)
  open circuit (pile) voltage/1(OCV_V) -> Add2/1, Product/1, charge loss/3(OCV_V), OCV_V/1
  charge loss/1(loss_pwr_W) -> Gain2/1
  Subtract1/1 -> Product1/2, Add2/2
  Integrator1/1 -> battery energy change/1
  Product/1 -> Gain5/1
  pile_curr_A/1 -> Product/2
  Rs/3(Rs_chg_Ohm) -> chg_res_Ohm/1
  Rs/2(Rs_dis_Ohm) -> dis_res_Ohm/1
  SoC_norm/1 -> Rs/1(SoC_norm), RC long term (LT)/1(SoC_norm), RC short term (ST)/1(SoC_norm), open circuit (pile) voltage/1(SoC_norm)
  Rs/1(Rs_V) -> Subtract1/3
  RC short term (ST)/1(RC_ST_V) -> Subtract1/1
  batt_temp_degC/1 -> Rs/3(batt_temp_degC), RC long term (LT)/3(batt_temp_degC), RC short term (ST)/3(batt_temp_degC), open circuit (pile) voltage/3(batt_temp_degC)
  RC long term (LT)/1(RC_LT_V) -> Subtract1/2
  Add2/1 -> batt_volts_V/1
  Add1/1 -> Integrator2/1, loss_pwr_W/1
  chg_eff_norm/1 -> charge loss/1(charge_eff_norm)
  Integrator3/1 -> battery energy discharge gross/1
  negative/1 -> Integrator3/1
  Gain5/1 -> negative/1, result integrator/1, Integrator1/1

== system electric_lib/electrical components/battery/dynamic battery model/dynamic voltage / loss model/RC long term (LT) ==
  SoC_norm : Inport
  cell_curr_A : Inport  Port=2
  batt_temp_degC : Inport  Port=3
  Add2 : Sum  Inputs=+-
  Cp long term : Subsystem
  Integrator : Integrator
  Product4 : Product  Inputs=*/
  Product5 : Product  Inputs=*/
  Rp long term : Subsystem
  use 2nd order : Gain  Gain=battery.use_second_order_model
  RC_LT_V : Outport
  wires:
  Rp long term/1(Rp_LT_Ohm) -> Product5/2
  batt_temp_degC/1 -> Cp long term/3(batt_temp_degC), Rp long term/3(batt_temp_degC)
  cell_curr_A/1 -> Cp long term/2(cell_curr_A), Rp long term/2(cell_curr_A), Add2/1
  SoC_norm/1 -> Cp long term/1(SoC_norm), Rp long term/1(SoC_norm)
  Integrator/1 -> Product5/1, use 2nd order/1
  Product4/1 -> Integrator/1
  Product5/1 -> Add2/2  "I LT"
  Add2/1 -> Product4/1
  Cp long term/1(Cp_LT_Farad) -> Product4/2
  use 2nd order/1 -> RC_LT_V/1

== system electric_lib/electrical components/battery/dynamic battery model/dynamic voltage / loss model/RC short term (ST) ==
  SoC_norm : Inport
  cell_curr_A : Inport  Port=2
  batt_temp_degC : Inport  Port=3
  Add2 : Sum  Inputs=+-
  Cp short term : Subsystem
  Integrator : Integrator
  Product4 : Product  Inputs=*/
  Product5 : Product  Inputs=*/
  Rp short term : Subsystem
  RC_ST_V : Outport
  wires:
  Cp short term/1(Cp_ST_Farad) -> Product4/2
  Add2/1 -> Product4/1
  Product5/1 -> Add2/2  "I ST"
  Product4/1 -> Integrator/1
  Integrator/1 -> RC_ST_V/1, Product5/1
  SoC_norm/1 -> Cp short term/1(SoC_norm), Rp short term/1(SoC_norm)
  cell_curr_A/1 -> Cp short term/2(cell_curr_A), Add2/1, Rp short term/2(cell_curr_A)
  batt_temp_degC/1 -> Cp short term/3(batt_temp_degC), Rp short term/3(batt_temp_degC)
  Rp short term/1(Rp_ST_Ohm) -> Product5/2

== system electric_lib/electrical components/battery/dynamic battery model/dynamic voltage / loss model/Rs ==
  SoC_norm : Inport
  cell_curr_A : Inport  Port=2
  batt_temp_degC : Inport  Port=3
  Product1 : Product
  Rs_chg : Lookup_n-D  BreakpointsForDimension1=battery.resistance_map_index_temp_degC  BreakpointsForDimension2=battery.resistance_map_index_soc_norm  Table=battery.resistance_map_charge_Ohms  RndMeth=Simplest
  Rs_dis : Lookup_n-D  BreakpointsForDimension1=battery.resistance_map_index_temp_degC  BreakpointsForDimension2=battery.resistance_map_index_soc_norm  Table=battery.resistance_map_discharge_Ohms  RndMeth=Simplest
  Switch : Switch  Criteria=u2 > Threshold
  Rs_V : Outport
  Rs_dis_Ohm : Outport  Port=2
  Rs_chg_Ohm : Outport  Port=3
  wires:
  Rs_chg/1 -> Rs_chg_Ohm/1, Switch/3
  Rs_dis/1 -> Switch/1, Rs_dis_Ohm/1
  SoC_norm/1 -> Rs_dis/2, Rs_chg/2
  batt_temp_degC/1 -> Rs_dis/1, Rs_chg/1
  cell_curr_A/1 -> Product1/1, Switch/2
  Switch/1 -> Product1/2
  Product1/1 -> Rs_V/1

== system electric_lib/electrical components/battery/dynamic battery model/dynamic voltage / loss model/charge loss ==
  charge_eff_norm : Inport
  cell_curr_A : Inport  Port=2
  OCV_V : Inport  Port=3
  Compare To Zero : simulink/Logic and Bit Operations/Compare To Zero  relop=<=  OutDataTypeStr=uint8
  Constant2 : Constant
  Data Type Conversion : DataTypeConversion  OutDataTypeStr=double
  Gain1 : Gain  Gain=-1
  Product7 : Product  Inputs=4  OutDataTypeStr=double
  Sum : Sum  Inputs=|+-
  loss_pwr_W : Outport
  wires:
  Product7/1 -> loss_pwr_W/1
  Sum/1 -> Product7/1
  Compare To Zero/1 -> Data Type Conversion/1
  Constant2/1 -> Sum/1
  Data Type Conversion/1 -> Product7/2
  charge_eff_norm/1 -> Sum/2
  OCV_V/1 -> Product7/4
  cell_curr_A/1 -> Compare To Zero/1, Gain1/1
  Gain1/1 -> Product7/3

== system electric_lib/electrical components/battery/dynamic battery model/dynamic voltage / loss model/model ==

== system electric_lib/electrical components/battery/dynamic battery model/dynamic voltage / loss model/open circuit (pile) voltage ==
  SoC_norm : Inport
  cell_curr_A : Inport  Port=2
  batt_temp_degC : Inport  Port=3
  OCV average : Lookup_n-D  BreakpointsForDimension1=battery.open_circuit_voltage_map_index_temp_degC  BreakpointsForDimension2=battery.open_circuit_voltage_map_index_soc_norm  Table=battery.open_circuit_voltage_map_average_V  RndMeth=Simplest
  OCV charge : Lookup_n-D  BreakpointsForDimension1=battery.open_circuit_voltage_map_index_temp_degC  BreakpointsForDimension2=battery.open_circuit_voltage_map_index_soc_norm  Table=battery.open_circuit_voltage_map_charge_V  RndMeth=Simplest
  OCV discharge : Lookup_n-D  BreakpointsForDimension1=battery.open_circuit_voltage_map_index_temp_degC  BreakpointsForDimension2=battery.open_circuit_voltage_map_index_soc_norm  Table=battery.open_circuit_voltage_map_discharge_V  RndMeth=Simplest
  Switch : Switch  Criteria=u2 ~= 0
  Switch1 : Switch
  use average : Constant  Value=battery.use_average_open_circuit_Volts
  OCV_V : Outport
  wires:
  use average/1 -> Switch/2
  Switch1/1 -> Switch/3
  OCV charge/1 -> Switch1/3
  OCV discharge/1 -> Switch1/1
  cell_curr_A/1 -> Switch1/2
  Switch/1 -> OCV_V/1
  OCV average/1 -> Switch/1
  batt_temp_degC/1 -> OCV discharge/1, OCV average/1, OCV charge/1
  SoC_norm/1 -> OCV charge/2, OCV discharge/2, OCV average/2

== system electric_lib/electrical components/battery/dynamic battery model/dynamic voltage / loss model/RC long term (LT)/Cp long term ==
  SoC_norm : Inport
  cell_curr_A : Inport  Port=2
  batt_temp_degC : Inport  Port=3
  Cp_LT_chg : Lookup_n-D  BreakpointsForDimension1=battery.transient_RC_index_temp_degC  BreakpointsForDimension2=battery.transient_RC_index_soc_norm  Table=battery.transient_C_charge_long_term_Farads  RndMeth=Simplest
  Cp_LT_dis : Lookup_n-D  BreakpointsForDimension1=battery.transient_RC_index_temp_degC  BreakpointsForDimension2=battery.transient_RC_index_soc_norm  Table=battery.transient_C_discharge_long_term_Farads  RndMeth=Simplest
  Switch : Switch
  Cp_LT_Farad : Outport
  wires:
  cell_curr_A/1 -> Switch/2
  Cp_LT_chg/1 -> Switch/3
  Cp_LT_dis/1 -> Switch/1
  Switch/1 -> Cp_LT_Farad/1
  SoC_norm/1 -> Cp_LT_chg/2, Cp_LT_dis/2
  batt_temp_degC/1 -> Cp_LT_chg/1, Cp_LT_dis/1

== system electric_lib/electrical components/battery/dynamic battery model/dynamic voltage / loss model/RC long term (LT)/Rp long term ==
  SoC_norm : Inport
  cell_curr_A : Inport  Port=2
  batt_temp_degC : Inport  Port=3
  Rp_LT_chg : Lookup_n-D  BreakpointsForDimension1=battery.transient_RC_index_temp_degC  BreakpointsForDimension2=battery.transient_RC_index_soc_norm  Table=battery.transient_R_charge_long_term_Ohms  RndMeth=Simplest
  Rp_LT_dis : Lookup_n-D  BreakpointsForDimension1=battery.transient_RC_index_temp_degC  BreakpointsForDimension2=battery.transient_RC_index_soc_norm  Table=battery.transient_R_discharge_long_term_Ohms  RndMeth=Simplest
  Switch : Switch
  Rp_LT_Ohm : Outport
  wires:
  cell_curr_A/1 -> Switch/2
  Rp_LT_chg/1 -> Switch/3
  Rp_LT_dis/1 -> Switch/1
  Switch/1 -> Rp_LT_Ohm/1
  SoC_norm/1 -> Rp_LT_chg/2, Rp_LT_dis/2
  batt_temp_degC/1 -> Rp_LT_chg/1, Rp_LT_dis/1

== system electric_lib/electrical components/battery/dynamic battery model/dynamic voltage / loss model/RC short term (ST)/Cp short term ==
  SoC_norm : Inport
  cell_curr_A : Inport  Port=2
  batt_temp_degC : Inport  Port=3
  Cp_ST_chg : Lookup_n-D  BreakpointsForDimension1=battery.transient_RC_index_temp_degC  BreakpointsForDimension2=battery.transient_RC_index_soc_norm  Table=battery.transient_C_charge_short_term_Farads  RndMeth=Simplest
  Cp_ST_dis : Lookup_n-D  BreakpointsForDimension1=battery.transient_RC_index_temp_degC  BreakpointsForDimension2=battery.transient_RC_index_soc_norm  Table=battery.transient_C_discharge_short_term_Farads  RndMeth=Simplest
  Switch : Switch
  Cp_ST_Farad : Outport
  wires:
  cell_curr_A/1 -> Switch/2
  Cp_ST_chg/1 -> Switch/3
  Cp_ST_dis/1 -> Switch/1
  Switch/1 -> Cp_ST_Farad/1
  SoC_norm/1 -> Cp_ST_chg/2, Cp_ST_dis/2
  batt_temp_degC/1 -> Cp_ST_chg/1, Cp_ST_dis/1

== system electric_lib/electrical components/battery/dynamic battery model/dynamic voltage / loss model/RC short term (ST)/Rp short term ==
  SoC_norm : Inport
  cell_curr_A : Inport  Port=2
  batt_temp_degC : Inport  Port=3
  Rp_ST_chg : Lookup_n-D  BreakpointsForDimension1=battery.transient_RC_index_temp_degC  BreakpointsForDimension2=battery.transient_RC_index_soc_norm  Table=battery.transient_R_charge_short_term_Ohms  RndMeth=Simplest
  Rp_ST_dis : Lookup_n-D  BreakpointsForDimension1=battery.transient_RC_index_temp_degC  BreakpointsForDimension2=battery.transient_RC_index_soc_norm  Table=battery.transient_R_discharge_short_term_Ohms  RndMeth=Simplest
  Switch : Switch
  Rp_ST_Ohm : Outport
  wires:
  cell_curr_A/1 -> Switch/2
  Rp_ST_chg/1 -> Switch/3
  Rp_ST_dis/1 -> Switch/1
  Switch/1 -> Rp_ST_Ohm/1
  SoC_norm/1 -> Rp_ST_chg/2, Rp_ST_dis/2
  batt_temp_degC/1 -> Rp_ST_chg/1, Rp_ST_dis/1
